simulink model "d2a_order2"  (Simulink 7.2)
settings: Solver=ode5  StartTime=0.0  StopTime=0.00005  FixedStep=1/(2*20000e5)  MaxStep=1/100e7  RelTol=1e-3  AbsTol=1e-6
undefined symbols (not defined in the file or in its folder): den, num

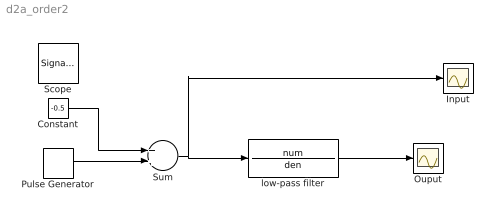
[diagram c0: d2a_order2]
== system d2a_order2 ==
  Constant : Constant  Value=-0.5  OutDataType=sfix(16)  OutScaling=2^0
  Input : Scope
  Ouput : Scope
  Pulse Generator : DiscretePulseGenerator  PulseType=Time based  Period=1/1000e3  PulseWidth=50
  Sum : Sum  OutDataType=sfix(16)  OutScaling=2^0
  low-pass filter : TransferFcn  Numerator=num  Denominator=den
  Scope : SignalViewerScope  IOType=viewer  ZoomMode=yonly  RefreshTime=0.035000
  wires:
  Sum/1 -> low-pass filter/1, Input/1
  Constant/1 -> Sum/1
  Pulse Generator/1 -> Sum/2
  low-pass filter/1 -> Ouput/1
